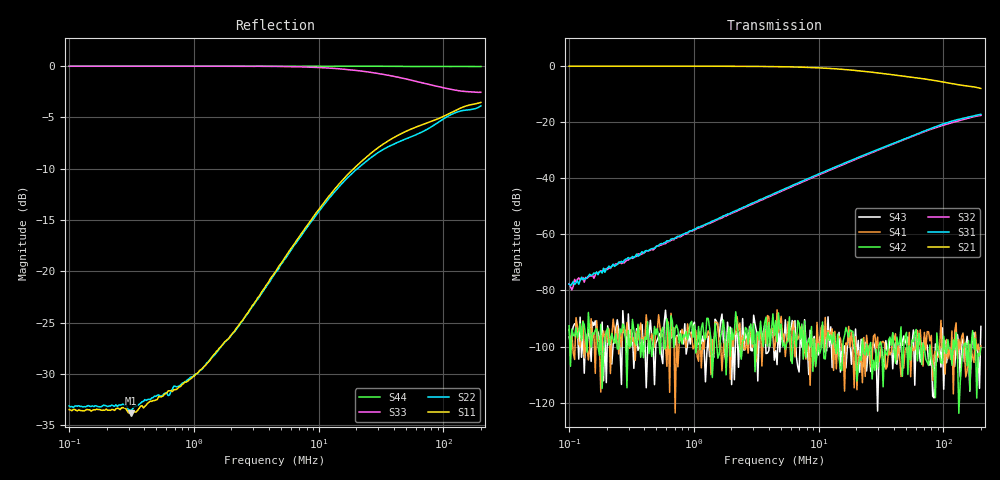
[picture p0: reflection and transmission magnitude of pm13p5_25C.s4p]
!Keysight Technologies,E5080A,MY55200740,A.12.60.03
!Date: Friday, October 02, 2020 16:13:59
!Correction: S11(Full 4 Port(1,2,3,4))
!S12(Full 4 Port(1,2,3,4))
!S13(Full 4 Port(1,2,3,4))
!S14(Full 4 Port(1,2,3,4))
!S21(Full 4 Port(1,2,3,4))
!S22(Full 4 Port(1,2,3,4))
!S23(Full 4 Port(1,2,3,4))
!S24(Full 4 Port(1,2,3,4))
!S31(Full 4 Port(1,2,3,4))
!S32(Full 4 Port(1,2,3,4))
!S33(Full 4 Port(1,2,3,4))
!S34(Full 4 Port(1,2,3,4))
!S41(Full 4 Port(1,2,3,4))
!S42(Full 4 Port(1,2,3,4))
!S43(Full 4 Port(1,2,3,4))
!S44(Full 4 Port(1,2,3,4))
!S4P File: Measurements: <S11,S12,S13,S14>,
!<S21,S22,S23,S24>,
!<S31,S32,S33,S34>,
!<S41,S42,S43,S44>:Log Frequency Sweep
# Hz S  dB  R 50
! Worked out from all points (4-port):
!   300 points, 100 kHz to 200 MHz, reference 50 ohm
!   strongest paths, dB at 100 kHz, 673 kHz, 4.529 MHz, 30.48 MHz, 200 MHz:
!     S21: -0.2, -0.2, -0.3, -2.6, -8.1
!     S31: -77.8, -61.6, -45.3, -29.7, -17.3
!     S32: -77.6, -61.9, -45.6, -30.0, -17.7
!     S42: -92.6, -91.1, -90.8, -99.7, -100.4
!     S41: -93.9, -96.6, -98.4, -105.4, -99.7
!     S43: -96.6, -95.0, -101.4, -103.7, -92.8
!   lowest |S11| = -33.8 dB at 313.9 kHz (marker M1), VSWR 1.04, Z = 52 - j0.416 ohm
!   |S11| at or under -10 dB: start of sweep to 19.09 MHz
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100000  -33.48 0.7  -0.19 -0.1  -78.04 98.2  -91.78 -76.7
        -0.19 -0.1  -33.13 1.0  -80.48 80.3  -91.81 99.0
        -77.78 83.1  -77.61 95.1  0.00 -0.1  -95.37 -176.7
        -93.86 136.6  -92.59 -161.6  -96.63 17.7  -0.00 -0.0
105215.7  -33.59 0.0  -0.19 -0.1  -77.36 90.6  -97.16 -66.5
          -0.19 -0.1  -33.18 -0.2  -77.72 96.8  -91.35 -141.4
          -77.79 84.0  -79.82 95.8  0.00 -0.1  -96.59 68.6
          -95.48 -98.8  -93.77 157.0  -95.14 -95.6  0.00 -0.0
313913.9  -33.85 -11.4  -0.19 -0.4  -68.52 88.8  -114.95 68.3
          -0.19 -0.4  -33.57 -11.1  -68.66 88.3  -100.50 128.4
          -68.55 88.7  -68.32 93.1  0.00 -0.4  -100.83 -53.8
          -94.00 -177.6  -99.75 99.9  -94.07 -81.9  -0.00 -0.0
1177342  -29.43 -56.2  -0.19 -1.5  -56.79 88.7  -92.27 167.4
         -0.19 -1.5  -29.48 -54.2  -57.08 88.8  -104.55 -163.7
         -56.92 88.3  -57.30 89.9  0.00 -1.4  -107.34 -116.1
         -98.52 -177.7  -91.57 30.0  -96.29 34.3  0.00 -0.1
2.13545e7  -9.44 -126.9  -1.85 -16.1  -32.44 78.0  -97.54 167.8
           -1.86 -16.1  -9.80 -116.3  -32.77 80.9  -96.95 -13.0
           -32.44 77.9  -32.77 81.0  -0.45 -23.8  -95.02 54.0
           -105.47 -71.0  -103.57 55.4  -109.15 37.6  -0.00 -1.5
8.215269e7  -5.34 -152.8  -5.16 -18.7  -22.10 61.3  -95.41 141.8
            -5.17 -18.7  -5.83 -131.5  -22.43 69.7  -101.00 0.2
            -22.10 61.3  -22.44 69.6  -1.86 -69.6  -100.41 52.8
            -112.10 170.3  -106.66 40.3  -117.68 134.6  -0.02 -5.6
2e8  -3.53 -163.4  -8.12 -9.7  -17.33 34.2  -107.98 4.6
     -8.12 -9.7  -3.87 -111.0  -17.73 57.3  -98.80 101.7
     -17.33 34.2  -17.72 57.4  -2.55 -114.1  -93.56 -59.8
     -99.75 -115.6  -100.36 127.3  -92.84 -44.2  -0.03 -13.5
